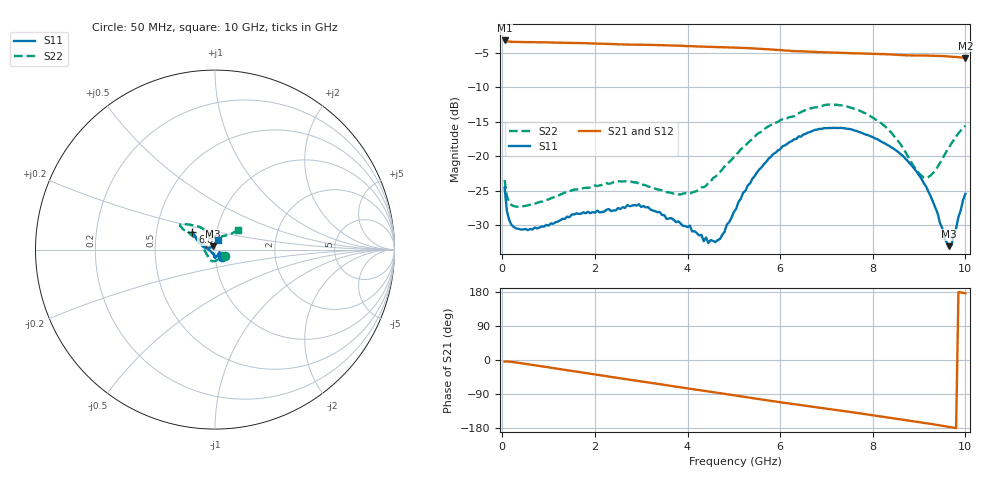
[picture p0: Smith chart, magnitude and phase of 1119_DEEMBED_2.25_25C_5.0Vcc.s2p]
!Hittite Microwave Corp.
!Digital Attenuator/PhaseShifter Rev 1.4.0
!Filename: C:\DATA\DATA\1119_DEEMBED_2.25_25C_5.0Vcc.s2p
!VNA ID: Agilent Technologies,N5224A,MY51441122,A.10.45.03
!Device type:
!2 Port Calibration.
!Temp(C): 25
!Lot Number:
!Serial Number:
!Operator:
!Misc:
!Attenuator:  2.250
# GHZ S DB R 50.0
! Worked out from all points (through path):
!   200 points, 50 MHz to 10 GHz, reference 50 ohm
!   highest |S21| = -3.16 dB at 50 MHz (marker M1); lowest = -5.7 dB at 10 GHz (marker M2)
!   group delay of S21, straight-line fit = 50.2 ps
!   lowest |S11| = -33.1 dB at 9.65 GHz (marker M3), VSWR 1.05, Z = 48.7 + j1.79 ohm
!   |S11| at or under -10 dB: start of sweep to end of sweep
!   |S22| runs from -27.4 to -12.5 dB; largest |S21 - S12| = 0.0017
!   S11 on the Smith chart (normalised r, x): 50 MHz: 1.08, -0.09; 6.85 GHz: 0.76, +0.15; 10 GHz: 1.03, +0.10
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0.05  -24.57 -45.3  -3.16 -4.1  -3.15 -4.1  -23.47 -34.6
0.1  -27.99 -38.9  -3.30 -3.8  -3.29 -3.8  -25.82 -28.8
0.15  -29.31 -34.1  -3.33 -4.3  -3.33 -4.3  -26.71 -25.2
0.3  -30.52 -29.1  -3.37 -6.5  -3.37 -6.6  -27.34 -24.2
1.75  -28.17 -80.2  -3.55 -33.5  -3.55 -33.5  -24.64 -74.5
2.75  -27.28 -88.4  -3.76 -51.9  -3.77 -51.9  -23.64 -108.5
3.4  -28.12 -95.0  -3.83 -63.8  -3.84 -63.8  -24.89 -131.5
4.05  -30.09 -101.1  -3.98 -75.7  -3.99 -75.8  -25.46 -161.4
4.45  -32.64 -127.1  -4.09 -83.0  -4.10 -83.1  -23.88 174.3
4.7  -32.05 -155.8  -4.14 -87.5  -4.16 -87.6  -22.33 161.6
5.05  -27.65 172.4  -4.21 -93.9  -4.22 -94.0  -19.77 151.8
5.2  -25.32 164.0  -4.25 -96.7  -4.27 -96.8  -18.71 149.9
5.75  -20.36 152.8  -4.45 -106.9  -4.47 -107.0  -15.65 147.7
6.7  -16.31 143.7  -4.81 -123.1  -4.82 -123.1  -12.98 146.3
6.85  -16.02 142.6  -4.86 -125.6  -4.88 -125.6  -12.82 146.0
7.65  -16.32 144.6  -5.03 -139.5  -5.04 -139.5  -13.20 139.6
8.35  -18.48 149.9  -5.19 -152.2  -5.19 -152.2  -16.21 124.6
9.1  -23.90 167.3  -5.35 -165.6  -5.36 -165.6  -23.08 91.5
9.3  -26.63 170.5  -5.37 -169.5  -5.39 -169.5  -22.46 71.9
9.65  -33.09 124.3  -5.49 -176.6  -5.51 -176.6  -18.67 46.3
9.7  -32.94 111.9  -5.52 -177.7  -5.53 -177.7  -18.14 44.6
10  -25.48 72.8  -5.69 176.2  -5.69 176.2  -15.58 40.6
